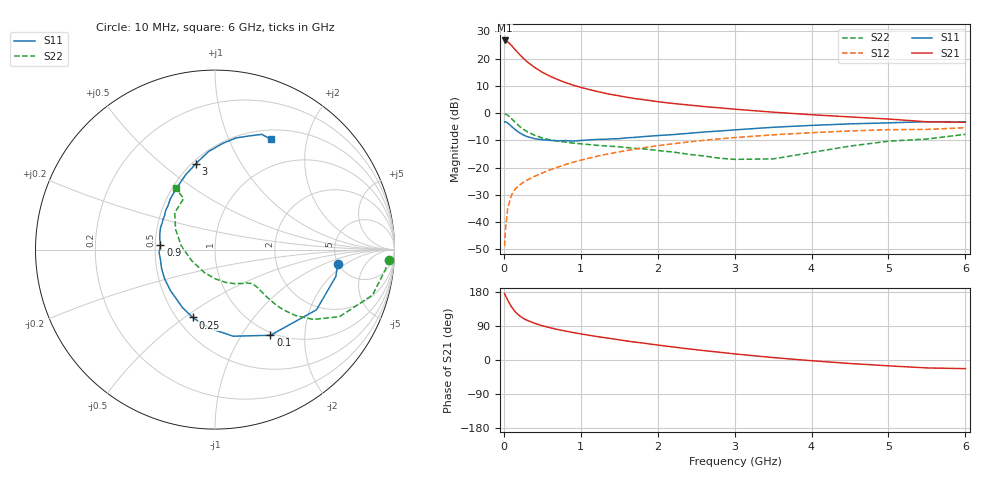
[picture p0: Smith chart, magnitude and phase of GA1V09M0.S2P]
! Infineon Technologies  Discrete & RF Semiconductors
! BF775
! Si NPN RF Bipolar Junction Transistor in SOT23
! VCE = 1 V  IC = 9 mA
! Common Emitter S-Parameters:  May  1996
# GHz  S  MA  R  50
!  f  S11  S21  S12  S22
! GHz  MAG  ANG  MAG  ANG  MAG  ANG  MAG  ANG
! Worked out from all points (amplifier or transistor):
!   36 points, 10 MHz to 6 GHz, reference 50 ohm
!   highest |S21| = 26.6 dB at 10 MHz (marker M1)
!   |S21| within 3 dB of that: start of sweep to 135.1 MHz
!   unconditionally stable (mu >= 1): 499 MHz to end of sweep
!   at 250 MHz: K = 0.70, MSG = 22.8 dB, |S12| = -25.5 dB
!   at 1.4 GHz: K = 1.17, MAG = 8.3 dB, |S12| = -14.8 dB
!   at 6 GHz: K = 1.03, MAG = 0.0 dB, |S12| = -5.4 dB
!   S11 on the Smith chart (normalised r, x): 10 MHz: 4.97, -1.47; 100 MHz: 0.96, -1.35; 250 MHz: 0.60, -0.54; 900 MHz: 0.53, +0.03; 3 GHz: 0.52, +0.66; 6 GHz: 0.62, +1.44
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0.01  0.6887 -6.5  21.48 175.5  0.0036 86.0  0.9713 -3.3
0.02  0.6897 -12.6  21.14 170.6  0.0069 84.6  0.9561 -6.6
0.05  0.6573 -30.7  20.29 157.9  0.0178 75.1  0.9136 -16.1
0.1  0.5685 -57.1  17.4 140.1  0.0314 66.0  0.7881 -28.3
0.15  0.493 -78.2  14.36 126.7  0.0406 59.9  0.6719 -35.4
0.2  0.4376 -94.6  12.07 117.3  0.0471 57.5  0.5775 -39.4
0.25  0.3981 -108.2  10.2 110.2  0.0531 56.6  0.5064 -41.4
0.3  0.3707 -119.2  8.789 104.9  0.0585 56.7  0.4583 -42.2
0.4  0.3373 -137.3  6.886 96.9  0.069 57.5  0.3916 -42.4
0.5  0.3242 -150.3  5.597 90.4  0.0792 58.8  0.3488 -42.1
0.6  0.3152 -160.9  4.742 85.2  0.0905 59.5  0.3228 -41.8
0.7  0.3092 -170.1  4.117 80.5  0.1014 60.0  0.3062 -41.8
0.9  0.3054 175.0  3.251 72.5  0.1249 59.9  0.2804 -42.7
1.1  0.3203 163.6  2.719 65.6  0.1479 59.2  0.2645 -45.3
1.3  0.3291 153.6  2.336 59.2  0.1713 57.8  0.25 -48.1
1.6  0.3509 141.6  1.945 50.1  0.2055 55.0  0.2321 -54.4
2.2  0.4017 122.5  1.497 34.4  0.2728 48.0  0.1925 -72.0
3  0.4903 102.6  1.176 16.1  0.3545 37.2  0.1411 -114.6
3.5  0.5475 93.8  1.037 6.4  0.3976 30.2  0.1437 -154.3
4.5  0.6327 79.4  0.848 -9.2  0.4689 16.5  0.2473 152.7
5.5  0.693 67.9  0.69 -20.9  0.4998 2.7  0.3334 121.6
6  0.6891 63.2  0.677 -22.8  0.5373 -1.1  0.4066 122.5
